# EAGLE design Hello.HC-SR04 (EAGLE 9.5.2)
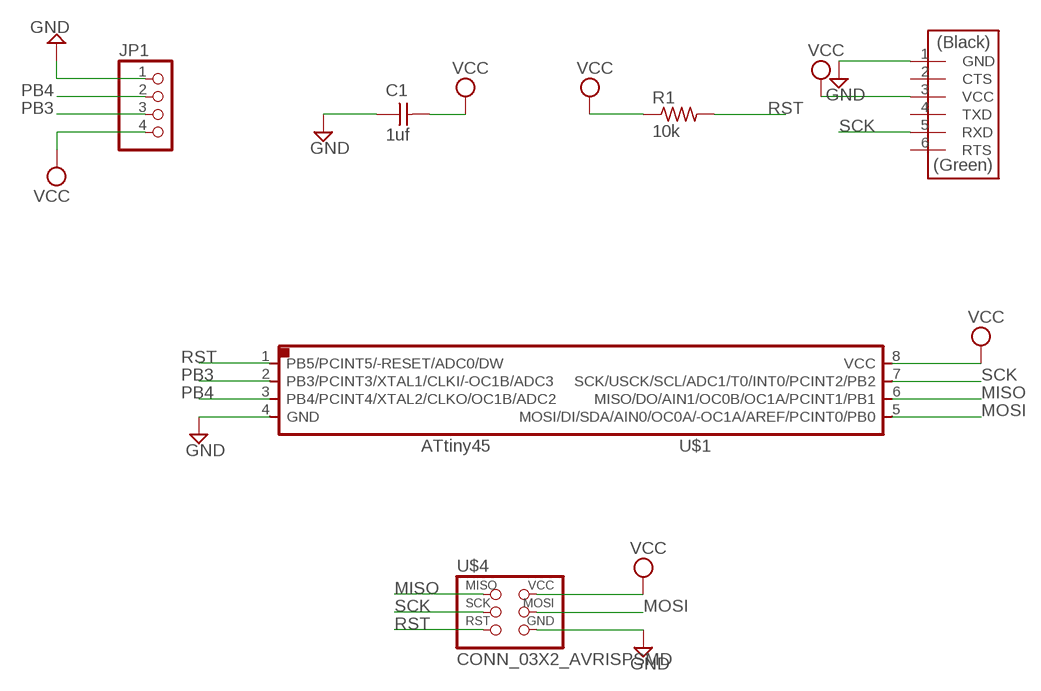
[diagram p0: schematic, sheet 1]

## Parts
C1  1uf  CAP_UNPOLARIZED  [C1206]
JP1  PINHD-1X4  [1X04]
R1  10k  R1206  [R1206]
U$1  UC_ATTINY45SI  [SOIC8]
U$3  CONN_06_FTDI-SMD-HEADER  [1X06SMD]
U$4  CONN_03X2_AVRISPSMD  [2X03SMD]

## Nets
GND: C1.1 JP1.1 U$1.4(GND) U$3.1(GND) U$4.6(GND)
MISO: U$1.6(MISO/DO/AIN1/OC0B/OC1A/PCINT1/PB1) U$4.1(MISO)
MOSI: U$1.5(MOSI/DI/SDA/AIN0/OC0A/-OC1A/AREF/PCINT0/PB0) U$4.4(MOSI)
PB3: JP1.3 U$1.2(PB3/PCINT3/XTAL1/CLKI/-OC1B/ADC3)
PB4: JP1.2 U$1.3(PB4/PCINT4/XTAL2/CLKO/OC1B/ADC2)
RST: R1.2 U$1.1(PB5/PCINT5/-RESET/ADC0/DW) U$4.5(RST)
SCK: U$1.7(SCK/USCK/SCL/ADC1/T0/INT0/PCINT2/PB2) U$3.5(RXD) U$4.3(SCK)
VCC: C1.2 JP1.4 R1.1 U$1.8(VCC) U$3.3(VCC) U$4.2(VCC)
Unconnected: U$3.2(CTS) U$3.4(TXD) U$3.6(RTS)

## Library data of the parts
C1 = fab:CAP_UNPOLARIZED
JP1 = pinhead:PINHD-1X4: PIN HEADER
R1 = fab:R: Resistor (US Symbol)
U$1 = fab:UC_ATTINY45
U$3 = fab:CONN_06_FTDI-SMD-HEADER
U$4 = fab:CONN_03X2_AVRISP

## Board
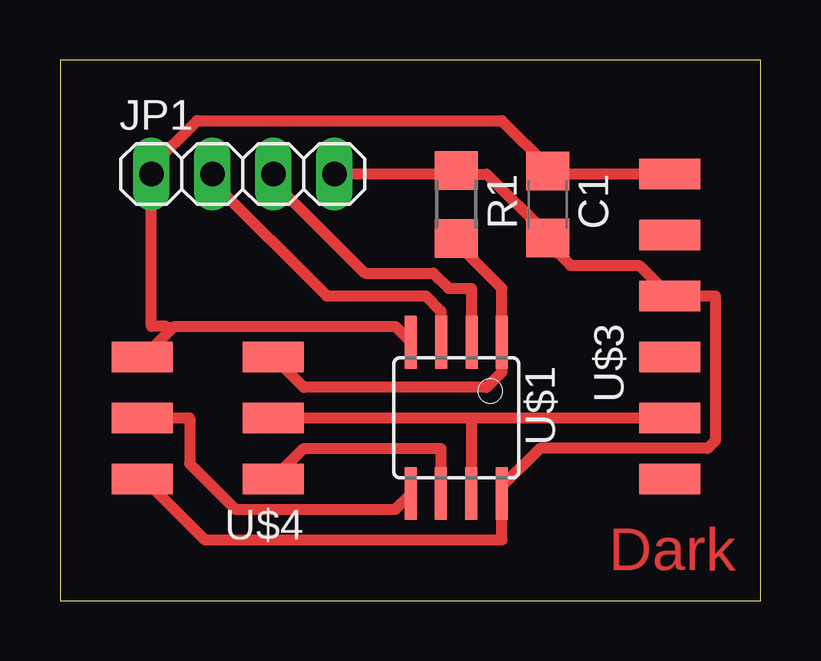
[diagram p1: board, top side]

Size 29.19 x 22.53 mm. Coordinates in mm from the lower left corner, seen from the top.
Outline: 0,0 29.19,0 29.19,22.53 0,22.53 0,0
Copper layers (1*16): Top 0.035mm / dielectric 1.5mm / Bottom 0.035mm
Design rules "fab-1": minimum track width 0.45mm, minimum drill 32mil, track to track 16mil, track to pad 16mil, pad to pad 16mil, via to via 16mil, smd to smd 6mil, copper to edge 16mil, drill to drill 16mil, minimum pad ring 10mil, minimum via ring 8mil, stop-mask expansion 4mil, vias tented up to drill 0mil, thermal gap 16mil

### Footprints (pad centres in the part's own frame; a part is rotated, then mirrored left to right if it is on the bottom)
C1206 = smd 1.6 x 1.8: 1 -1.4,0; 2 1.4,0
1X04 = drill 1.016 long: 1 -3.81,0; 2 -1.27,0; 3 1.27,0; 4 3.81,0
R1206 = smd 1.6 x 1.803: 1 -1.422,0; 2 1.422,0
SOIC8 = smd 0.5 x 2.2: 1 -1.905,-3.154; 2 -0.645,-3.154; 3 0.625,-3.154; 4 1.895,-3.154; 5 1.905,3.154; 6 0.635,3.154; 7 -0.635,3.154; 8 -1.905,3.154
1X06SMD = smd 2.54 x 1.27: 1 0,6.35; 2 0,3.81; 3 0,1.27; 4 0,-1.27; 5 0,-3.81; 6 0,-6.35
2X03SMD = smd 2.54 x 1.27: 1 -2.54,2.54; 2 2.92,2.54; 3 -2.54,0; 4 2.92,0; 5 -2.54,-2.54; 6 2.92,-2.54

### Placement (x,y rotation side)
C1  20.32,16.51 270 top
JP1  7.62,17.78 0 top
R1  16.51,16.51 270 top
U$1  16.51,7.62 180 top
U$3  25.4,11.43 0 top
U$4  6.35,7.62 180 top

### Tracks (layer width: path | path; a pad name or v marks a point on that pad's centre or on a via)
GND
  Top 0.45: U$3.1 20.32,17.78 C1.1 20.32,18.1 18.41,20 5.71,20 3.81,18.1 JP1.1 3.81,11.43 4.44,11.43 4.6,11.27 | 4.6,11.27 3.49,10.16 U$4.6 | 4.6,11.27 4.76,11.43 13.97,11.43 14.6,10.8 U$1.4
MISO
  Top 0.45: U$1.6 15.87,6.35 10.16,6.35 U$4.1
MOSI
  Top 0.45: U$4.4 5.4,7.62 5.4,5.72 7.3,3.81 13.97,3.81 14.6,4.45 U$1.5
PB3
  Top 0.45: JP1.3 8.89,17.46 12.7,13.65 15.56,13.65 16.19,13.02 17.14,13.02 17.14,10.8 U$1.2
PB4
  Top 0.45: JP1.2 6.35,17.46 11.11,12.7 15.24,12.7 15.87,12.07 15.87,10.8 U$1.3
RST
  Top 0.45: R1.2 16.51,14.92 18.41,13.02 U$1.1 18.41,9.52 17.78,8.89 10.16,8.89 U$4.5
SCK
  Top 0.45: 17.14,7.62 U$1.7 | U$4.3 17.14,7.62 | 17.14,7.62 U$3.5
VCC
  Top 0.45: U$4.2 3.49,5.08 6.03,2.54 18.41,2.54 U$1.8 18.41,4.76 20,6.35 26.99,6.35 27.3,6.67 27.3,12.7 U$3.3 24.13,13.97 21.27,13.97 20.32,14.92 C1.2 20.32,15.24 17.78,17.78 16.51,17.78 | 16.51,17.78 JP1.4 | 16.51,17.78 R1.1

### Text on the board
Top: Dark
